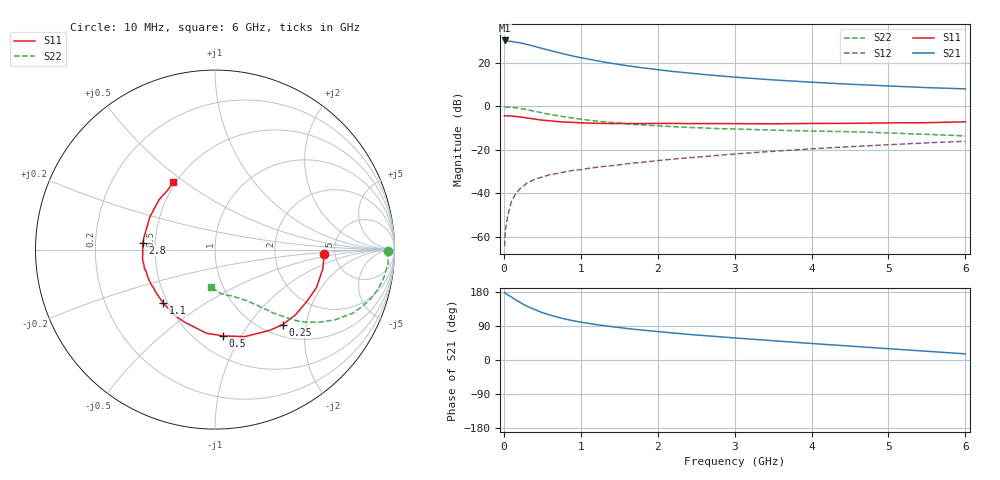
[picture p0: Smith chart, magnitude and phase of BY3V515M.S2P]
! SIEMENS Small Signal Semiconductors
! BFY420
! Si NPN RF SIEGET Grounded Emitter Transistor in MICRO-X
! VCE = 3.5 V  IC = 15 mA
! Common Emitter S-Parameters:  October  1996
# GHz  S  MA  R  50
!  f  S11  S21  S12  S22
! GHz  MAG  ANG  MAG  ANG  MAG  ANG  MAG  ANG
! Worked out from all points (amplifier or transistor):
!   36 points, 10 MHz to 6 GHz, reference 50 ohm
!   highest |S21| = 30.5 dB at 10 MHz (marker M1)
!   |S21| within 3 dB of that: start of sweep to 428 MHz
!   unconditionally stable (mu >= 1): start of sweep to 13.86 MHz; 2.238 GHz to end of sweep
!   at 250 MHz: K = 0.27, MSG = 32.9 dB, |S12| = -36.8 dB
!   at 1.4 GHz: K = 0.85, MSG = 23.6 dB, |S12| = -27.3 dB
!   at 6 GHz: K = 1.07, MAG = 10.4 dB, |S12| = -16.1 dB
!   S11 on the Smith chart (normalised r, x): 10 MHz: 4.06, -0.30; 250 MHz: 1.21, -1.48; 500 MHz: 0.67, -0.84; 1.1 GHz: 0.47, -0.34; 2.8 GHz: 0.43, +0.04; 6 GHz: 0.48, +0.45
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0.01  0.6063 -2.2  33.31 178.5  0.0006 62.2  0.9654 -0.6
0.02  0.6081 -4.0  33.09 175.9  0.0014 63.4  0.9633 -1.5
0.05  0.6104 -10.0  32.08 172.0  0.003 75.0  0.9682 -4.4
0.1  0.6035 -20.5  31.57 166.1  0.0066 77.2  0.9541 -9.2
0.15  0.5879 -29.3  30.52 158.8  0.0094 73.9  0.9346 -13.7
0.2  0.5771 -39.1  29.59 153.4  0.0122 72.2  0.9091 -17.6
0.25  0.5626 -48.0  28.33 147.3  0.0144 68.4  0.8764 -21.4
0.3  0.5434 -55.9  26.95 142.1  0.0171 66.8  0.8451 -24.8
0.4  0.5124 -71.1  24.36 133.4  0.0208 63.0  0.7765 -30.2
0.5  0.4829 -84.6  21.7 124.9  0.0237 60.3  0.713 -34.5
0.6  0.4684 -95.9  19.57 118.6  0.0268 57.0  0.6592 -37.9
0.8  0.4374 -113.8  15.96 108.0  0.0312 55.6  0.5721 -42.6
0.9  0.4293 -120.9  14.53 103.6  0.0335 55.1  0.5382 -44.1
1.1  0.4149 -133.9  12.37 96.6  0.0374 55.3  0.4846 -47.1
1.3  0.4069 -144.0  10.61 90.8  0.0415 55.3  0.4439 -49.1
1.6  0.4043 -155.8  8.721 83.1  0.0475 55.1  0.3983 -52.2
2.2  0.4073 -172.6  6.417 71.3  0.0611 54.3  0.344 -57.4
2.8  0.4034 174.5  5.092 61.3  0.075 52.5  0.3077 -62.1
3.5  0.3993 161.9  4.1 50.9  0.0925 48.9  0.2846 -67.5
4.5  0.4084 145.5  3.256 36.7  0.1181 41.9  0.2621 -76.1
5.5  0.4227 128.8  2.723 23.0  0.1448 33.6  0.2272 -88.6
6  0.4428 121.8  2.546 16.2  0.1574 29.1  0.2097 -96.7
